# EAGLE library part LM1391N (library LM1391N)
IC PHASE-LOCKED LOOP 8DIP Source: Datasheet
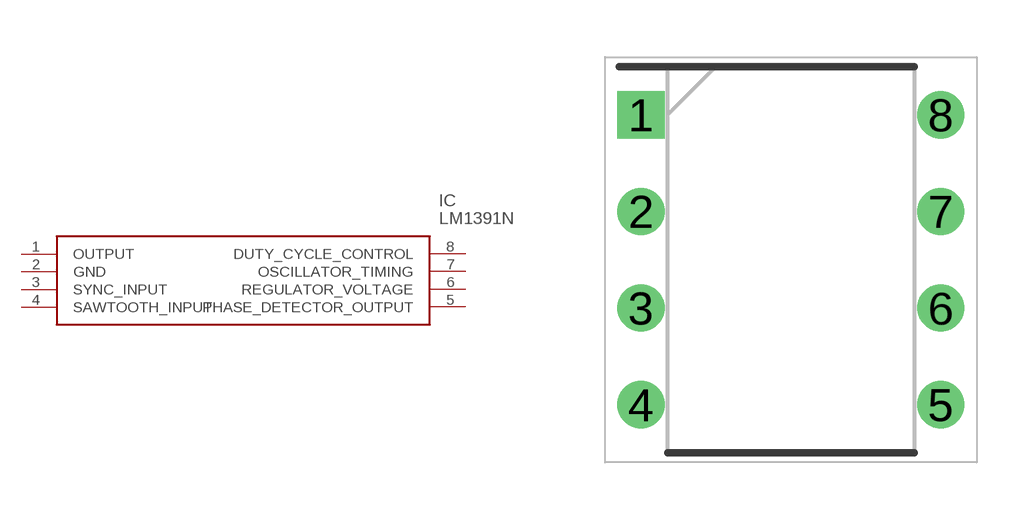
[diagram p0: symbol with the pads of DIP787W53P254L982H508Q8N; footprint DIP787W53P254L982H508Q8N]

Designator prefix IC

## LM1391N (Description: IC PHASE-LOCKED LOOP 8DIP; Height: 5.08mm; Manufacturer_Name: Texas Instruments; Manufacturer_Part_Number: LM1391N)  [DIP787W53P254L982H508Q8N]
1  OUTPUT
2  GND
3  SYNC_INPUT
4  SAWTOOTH_INPUT
5  PHASE_DETECTOR_OUTPUT
6  REGULATOR_VOLTAGE
7  OSCILLATOR_TIMING
8  DUTY_CYCLE_CONTROL

## Footprint DIP787W53P254L982H508Q8N (pad centres in mm)
DS75176BN
drill 0.733 pad 1.133 square: 1 -3.937,3.81
drill 0.733 pad 1.133: 2 -3.937,1.27; 3 -3.937,-1.27; 4 -3.937,-3.81; 5 3.937,-3.81; 6 3.937,-1.27; 7 3.937,1.27; 8 3.937,3.81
